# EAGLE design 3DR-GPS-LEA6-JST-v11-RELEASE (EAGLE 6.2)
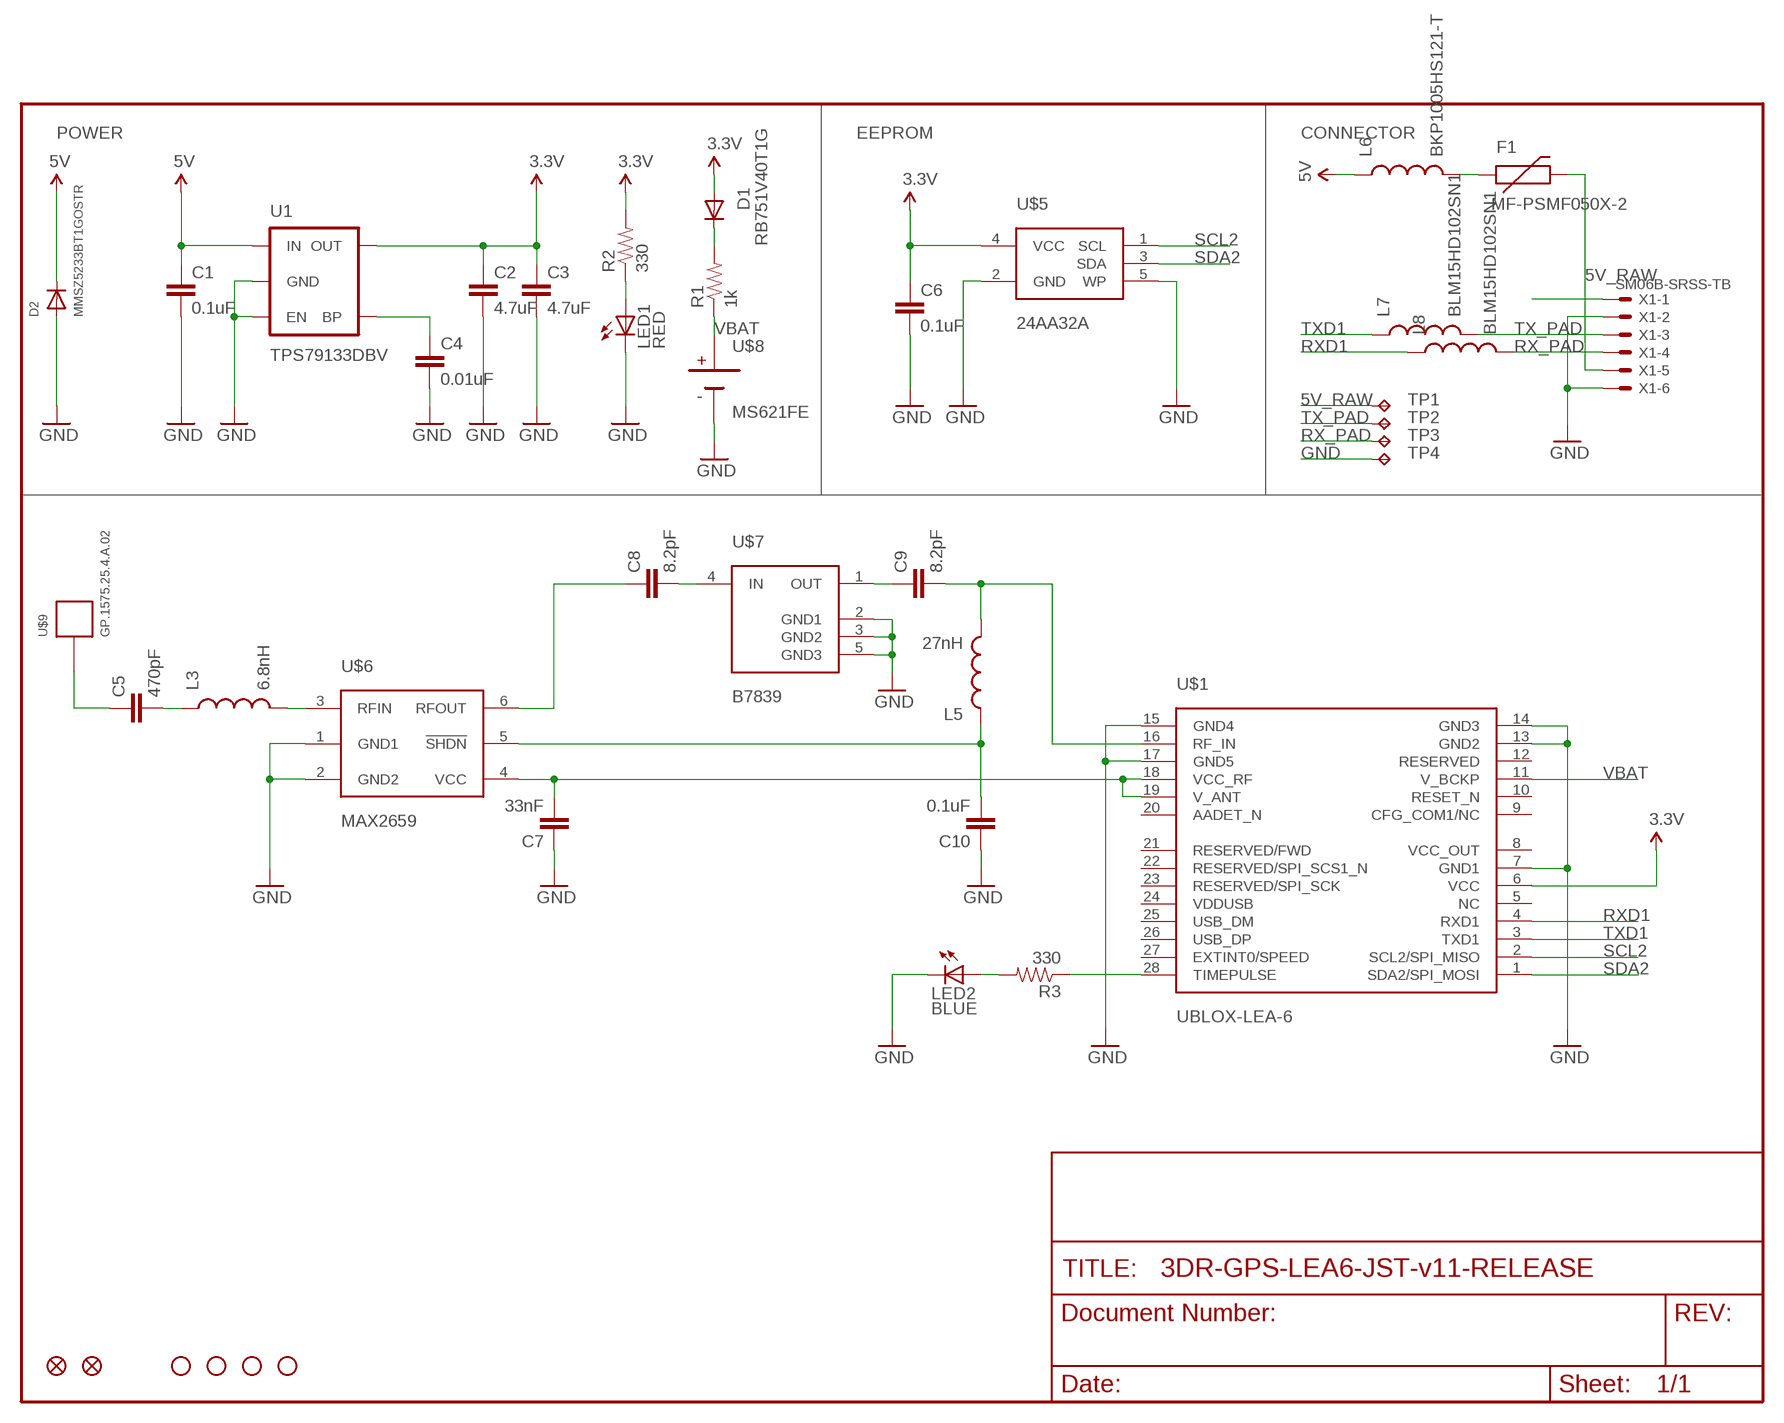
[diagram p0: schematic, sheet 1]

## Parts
C1  0.1uF  CAP0402-CAP  [0402-CAP]
C2  4.7uF  CAP0805  [0805]
C3  4.7uF  CAP0805  [0805]
C4  0.01uF  CAP0402-CAP  [0402-CAP]
C5  470pF  CAP0402-CAP  [0402-CAP]
C6  0.1uF  CAP0402-CAP  [0402-CAP]
C7  33nF  CAP0402-CAP  [0402-CAP]
C8  8.2pF  CAP0402-CAP  [0402-CAP]
C9  8.2pF  CAP0402-CAP  [0402-CAP]
C10  0.1uF  CAP0402-CAP  [0402-CAP]
D1  RB751V40T1G  DIODESOD  [SOD-323]
D2  MMSZ5233BT1GOSTR  DIODESOD-123  [SOD-123]
F1  MF-PSMF050X-2  PTC  [0805]
JP1  FIDUCIAL1X2  [FIDUCIAL-1X2]
JP2  FIDUCIAL1X2  [FIDUCIAL-1X2]
JP3  STAND-OFF  [STAND-OFF]
JP4  STAND-OFF  [STAND-OFF]
JP5  STAND-OFF  [STAND-OFF]
JP6  STAND-OFF  [STAND-OFF]
L3  6.8nH  INDUCTOR0402  [C0402]
L5  27nH  INDUCTOR0402  [C0402]
L6  BKP1005HS121-T  INDUCTOR0402  [0402-IND]
L7  BLM15HD102SN1  INDUCTOR0402  [0402-IND]
L8  BLM15HD102SN1  INDUCTOR0402  [0402-IND]
LED1  RED  LED0603  [LED-0603]
LED2  BLUE  LED0603  [LED-0603]
R1  1k  RESISTOR0402-RES  [0402-RES]
R2  330  RESISTOR0402-RES  [0402-RES]
R3  330  RESISTOR0402-RES  [0402-RES]
TP1  TPTP20SQ  [TP20SQ]
TP2  TPTP20SQ  [TP20SQ]
TP3  TPTP20SQ  [TP20SQ]
TP4  TPTP20SQ  [TP20SQ]
U1  TPS79133DBV  V_REG_LDOSMD  [SOT23-5]
U$1  UBLOX-LEA-6  [UBLOX-LEA-6]
U$5  24AA32A  [SOT23-5]
U$6  MAX2659  [UDFN-6]
U$7  B7839  [QCS5E]
U$8  MS621FE  [MS621FE]
U$9  GP.1575.25.4.A.02  [GP.1575.25.4.A.02]
X1  SM06B-SRSS-TB  [SM06B-SRSS-TB]

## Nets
3.3V: C2.1 C3.1 C6.1 D1.2(A) R2.2 U1.5(OUT) U$1.6(VCC) U$5.4(VCC)
5V: C1.1 D2.C L6.1 U1.1(IN)
5V_RAW: F1.2 TP1.TP X1.5
GND: C1.2 C2.2 C3.2 C4.2 C6.2 C7.1 C10.1 D2.A LED1.C LED2.C TP4.TP U1.2(GND) U1.3(EN) U$1.7(GND1) U$1.13(GND2) U$1.14(GND3) U$1.15(GND4) U$1.17(GND5) U$5.2(GND) U$5.5(WP) U$6.1(GND1) U$6.2(GND2) U$7.2(GND1) U$7.3(GND2) U$7.5(GND3) U$8.2(NEG) X1.2 X1.6
N$1: L3.2 U$6.3(RFIN)
N$2: C4.1 U1.4(BP)
N$3: C5.2 L3.1
N$4: C8.2 U$7.4(IN)
N$5: R3.1 U$1.28(TIMEPULSE)
N$6: C9.1 U$7.1(OUT)
N$7: C7.2 U$1.18(VCC_RF) U$1.19(V_ANT) U$6.4(VCC)
N$8: C8.1 U$6.6(RFOUT)
N$9: C10.2 L5.1 U$6.5(!SHDN)
N$10: C5.1 U$9.1(PIN)
N$11: C9.2 L5.2 U$1.16(RF_IN)
N$12: D1.1(C) R1.2
N$13: LED1.A R2.1
N$14: X1.1
N$15: LED2.A R3.2
N$16: F1.1 L6.2
RX_PAD: L8.2 TP3.TP X1.4
RXD1: L8.1 U$1.4(RXD1)
SCL2: U$1.2(SCL2/SPI_MISO) U$5.1(SCL)
SDA2: U$1.1(SDA2/SPI_MOSI) U$5.3(SDA)
TX_PAD: L7.2 TP2.TP X1.3
TXD1: L7.1 U$1.3(TXD1)
VBAT: R1.1 U$1.11(V_BCKP) U$8.1(POS)
Unconnected: U$1.5(NC) U$1.8(VCC_OUT) U$1.9(CFG_COM1/NC) U$1.10(RESET_N) U$1.12(RESERVED) U$1.20(AADET_N) U$1.21(RESERVED/FWD) U$1.22(RESERVED/SPI_SCS1_N) U$1.23(RESERVED/SPI_SCK) U$1.24(VDDUSB) U$1.25(USB_DM) U$1.26(USB_DP) U$1.27(EXTINT0/SPEED)

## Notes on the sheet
- POWER | EEPROM | CONNECTOR

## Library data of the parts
C1-C10 = SparkFun:CAP: Capacitor
D1 = SparkFun:DIODE: Diode
D2 = adafruit:DIODE: Diode
F1 = 3DRobotics:PTC: Resettable Fuse PTC; DATASHEET: http://www.bourns.com/data/global/PDFs/mfpsmf.pdf; LINK: http://parts.digikey.com/1/parts/1323493-fuse-ptc-resettable-smd-0805-mf-psmf050x-2.html; MFGPN: MF-PSMF050X-2
JP1 JP2 = SparkFun:FIDUCIAL: Fiducial Alignment Points
JP3-JP6 = SparkFun:STAND-OFF: Stand Off
L3 L5 = SparkFun:INDUCTOR: Inductors
L6-L8 = pixhawk2:INDUCTOR: Inductors
LED1 LED2 = SparkFun:LED: LEDs
R1-R3 = SparkFun:RESISTOR: Resistor
TP1-TP4 = testpad:TP: Test pad
U1 = SparkFun:V_REG_LDO: Voltage Regulator LDO Standard 150mA LDO voltage regulator in SOT-23 layout. Micrel part MIC5205. BP (by-pass) pin is used to lower output noise with 470pF cap.
U$1 = 3DRobotics:UBLOX-LEA-6: u-blox LEA-6 GPS Module The LEA-6 module series is a family of stand-alone GPS receivers featuring the high performance u-blox 6 positioning engine. These versatile receivers feature an extensive and flexible range of functionality, connectivity and cost savings options. LEA-6 modules maintain the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; DATASHEET: http://www.u-blox.com/images/downloads/Product_Docs/LEA-6_DataSheet_%28GPS.G6-HW-09004%29.pdf; LINK: http://www.u-blox.com/en/gps-modules/pvt-modules/lea-6-family.html; MFGPN: LEA-6
U$5 = 3DRobotics:24AA32A: Microchip 24AA32A 32K I2C EEPROM The Microchip Technology Inc. 24AA32A/24LC32A (24XX32A*) is a 32 Kbit Electrically Erasable PROM. The device is organized as a single block of 4K x 8-bit memory with a 2-wire serial interface. Low-voltage design permits operation down to 1.7V, with standby and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; DATASHEET: http://ww1.microchip.com/downloads/en/DeviceDoc/21713L.pdf; LINK: http://www.microchip.com/wwwproducts/Devices.aspx?dDocName=en010787; MFGPN: 24AA32A
U$6 = 3DRobotics:MAX2659: MAX2659 GPS/GNSS Low-Noise Amplifier The MAX2659 high-gain, low-noise amplifier (LNA) is designed for GPS, Galileo, and GLONASS applications. Designed in Maxim?s advanced SiGe process, the device achieves a 20.5dB gain and an ultra-low-noise figure of 0.8dB while maximizing the input-referred 1dB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; DATASHEET: http://datasheets.maxim-ic.com/en/ds/MAX2659.pdf; LINK: http://www.maxim-ic.com/datasheet/index.mvp/id/5299; MFGPN: MAX2659
U$7 = 3DRobotics:B7839: EPCOS B7839 SAW Rx Filter; DATASHEET: http://www.epcos.com/inf/40/ds/mc/B7839.pdf; MFGPN: B7839
U$8 = 3DRobotics:MS621FE: SEIKO 6.8mm Rechargeable 3V lithium battery; DATASHEET: http://speed.sii.co.jp/data/file_PRODUCT_MASTER_50112_TITLE_IMAGESP.pdf; LINK: http://search.digikey.com/us/en/products/MS621FE-FL11E/728-1057-ND/1889208; MFGPN: MS621FE
U$9 = 3DRobotics:GP.1575.25.4.A.02: Taoglas GP.1575.25.4.A.02 4mm thick GPS Patch Antenna, 1575MHz; DATASHEET: http://www.taoglas.com/images/product_images/original_images/GP.1575.25.4.A.02%20GPS%20Patch%20Antenna%201575MHz%20190410.pdf; LINK: http://www.taoglas.com/antennas/GPS-GLONASS_Antennas/Internal_GPS_-_Passive_Ceramic_Patch_Antennas/; MFGPN: GP.1575.25.4.A.02
X1 = con-jst2:?M06B-SRSS-TB: Disconnectable Crimp style connector, 1.0mm pitch 6 contacts

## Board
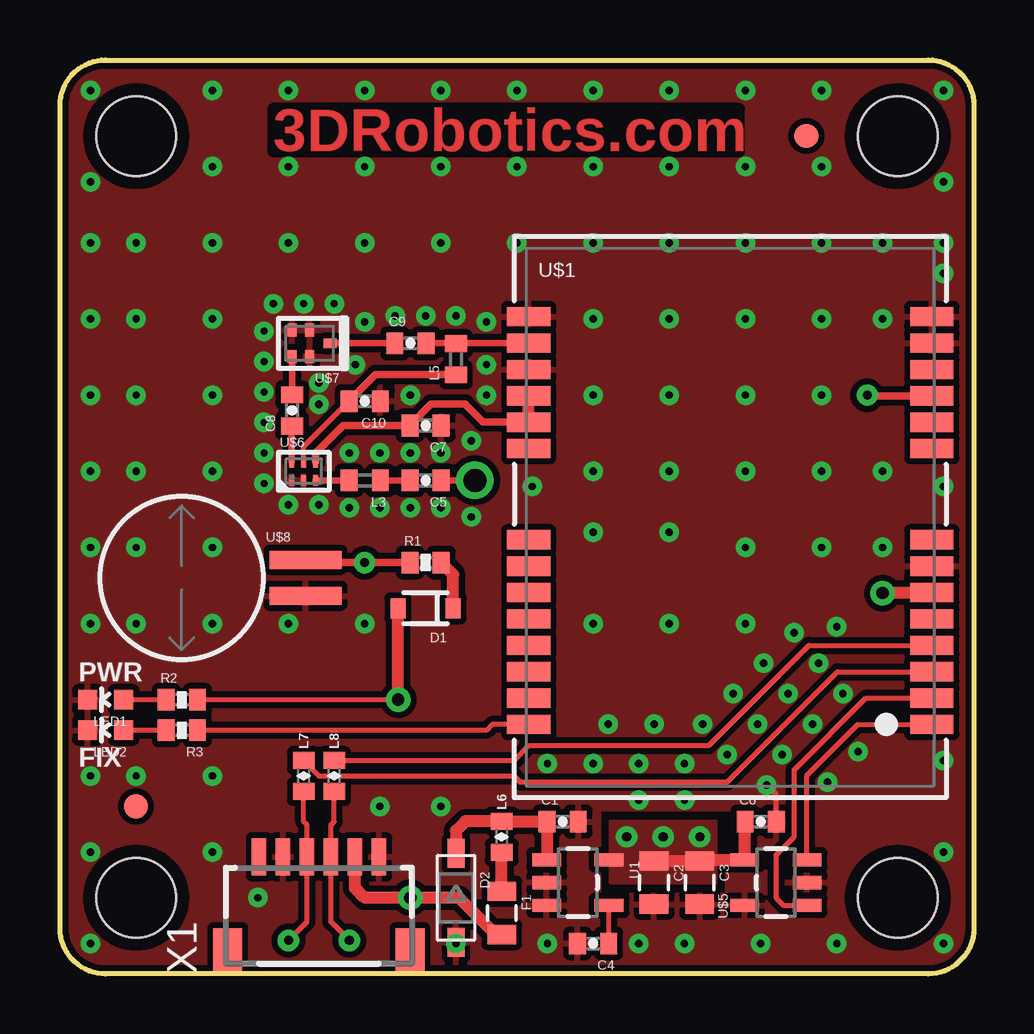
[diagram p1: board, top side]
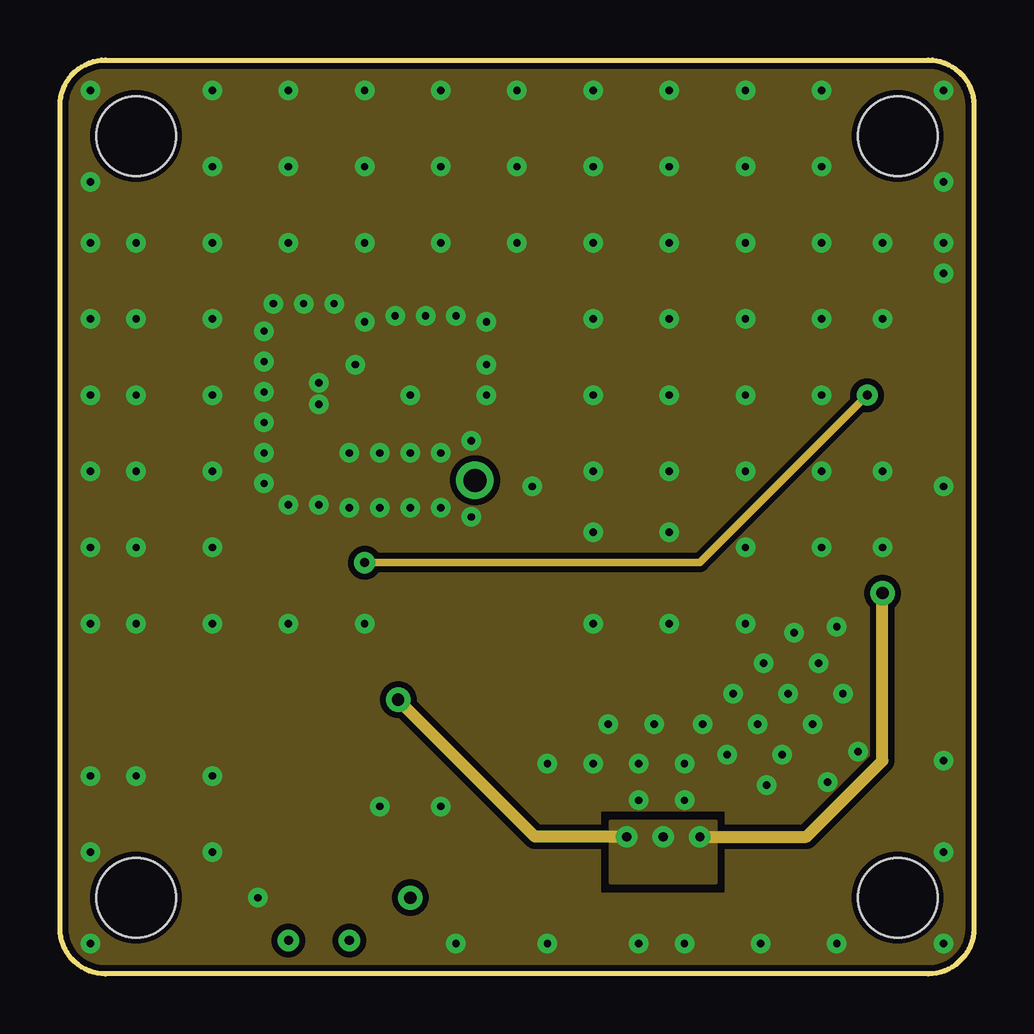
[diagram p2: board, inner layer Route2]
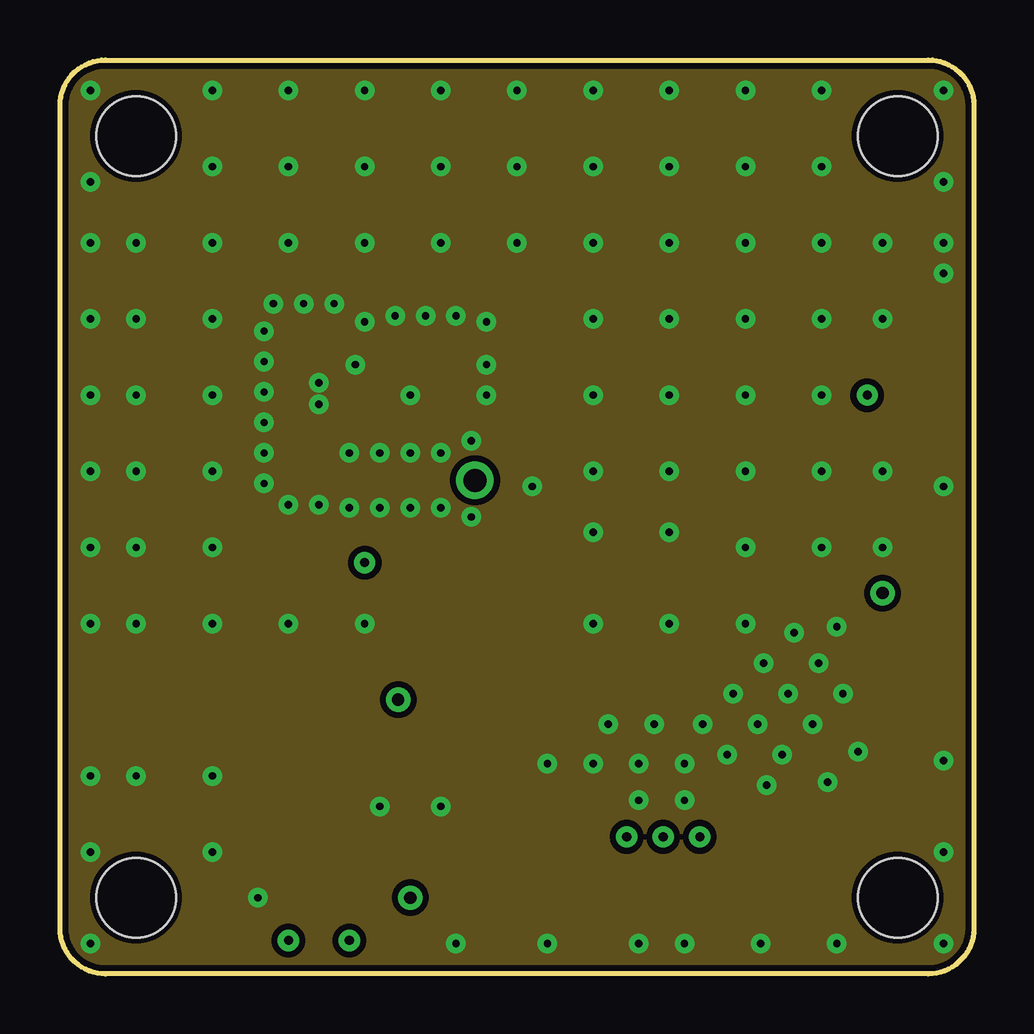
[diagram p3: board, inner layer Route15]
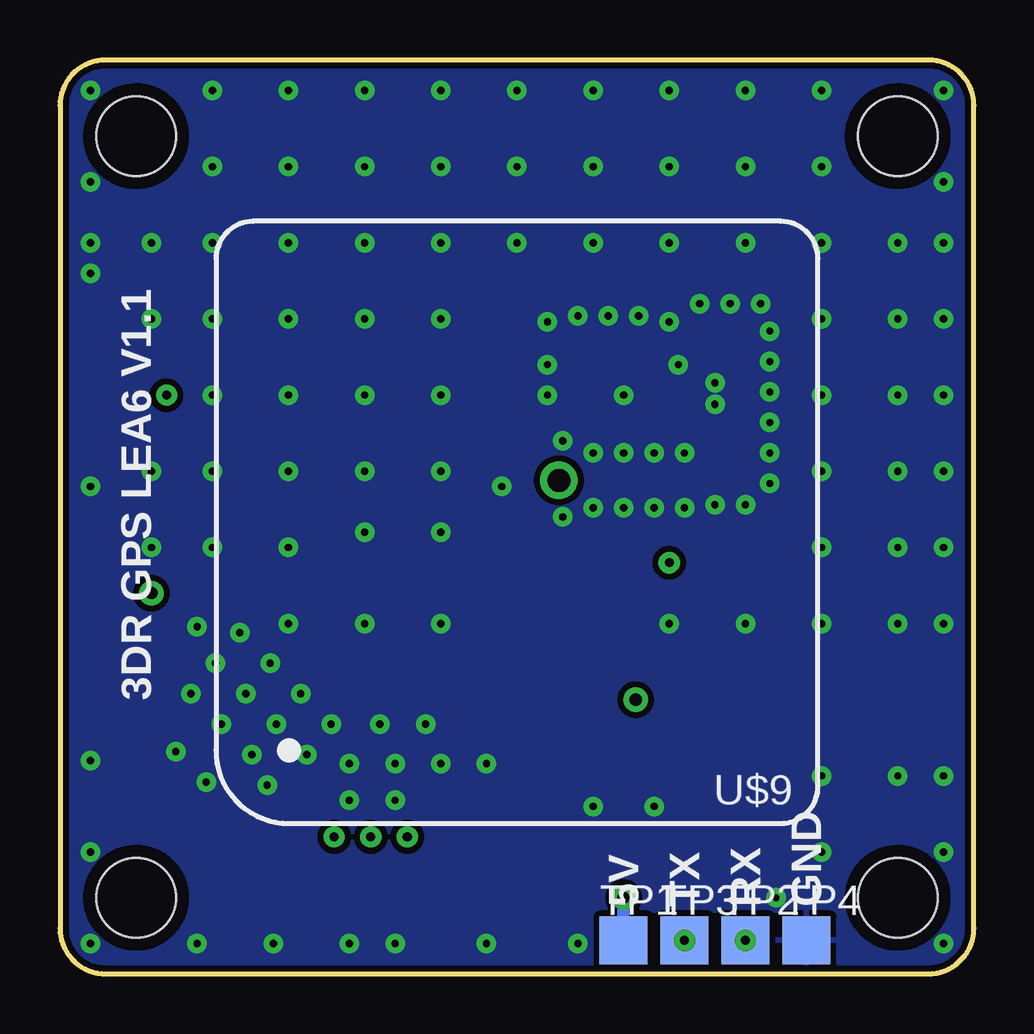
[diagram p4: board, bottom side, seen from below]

Size 38.1 x 38.1 mm. Coordinates in mm from the lower left corner, seen from the top.
Outline: 1.91,0 arc-90 0,1.91 0,36.2 arc-90 1.91,38.1 36.2,38.1 arc-90 38.1,36.2 38.1,1.91 arc-90 36.2,0 1.91,0
Copper layers (1*2*15*16): Top 0.035mm / dielectric 0.5mm / Route2 0.035mm / dielectric 0.5mm / Route15 0.035mm / dielectric 0.5mm / Bottom 0.035mm
Design rules: minimum track width 7mil, minimum drill 10mil, track to track 7mil, track to pad 7mil, pad to pad 7mil, via to via 7mil, smd to smd 0mil, copper to edge 10mil, drill to drill 8mil, minimum pad ring 12mil, minimum via ring 10mil, stop-mask expansion 4mil, vias tented up to drill 25mil, thermal gap 10mil

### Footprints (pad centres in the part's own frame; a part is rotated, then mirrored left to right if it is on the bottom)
0402-CAP = smd 0.7 x 0.9: 1 -0.65,0; 2 0.65,0
0805 = smd 0.8 x 1.2: 1 -0.9,0; 2 0.9,0
SOD-323 = smd 0.63 x 0.83: 1 -1.15,0; 2 1.15,0
SOD-123 = smd 1.2 x 0.7: A 1.85,0; C -1.85,0
FIDUCIAL-1X2 = smd 1 x 1: 1 0,0
STAND-OFF = hole 3.302: 0,0
C0402 = smd 0.7 x 0.9: 1 -0.65,0; 2 0.65,0
0402-IND = smd 0.7 x 0.9: 1 -0.65,0; 2 0.65,0
LED-0603 = smd 0.8 x 0.8: A 0,-0.75; C 0,0.75
0402-RES = smd 0.7 x 0.9: 1 -0.65,0; 2 0.65,0
TP20SQ = smd 2 x 2: TP 0,0
SOT23-5 = smd 0.55 x 1.2: 1 -0.95,-1.3; 2 0,-1.3; 3 0.95,-1.3; 4 0.95,1.3; 5 -0.95,1.3
UBLOX-LEA-6 = smd 1.8 x 0.8: 1 8.4,-8.65; 2 8.4,-7.55; 3 8.4,-6.45; 4 8.4,-5.35; 5 8.4,-4.25; 6 8.4,-3.15; 7 8.4,-2.05; 8 8.4,-0.95; 9 8.4,2.85; 10 8.4,3.95; 11 8.4,5.05; 12 8.4,6.15; 13 8.4,7.25; 14 8.4,8.35; 15 -8.4,8.35; 16 -8.4,7.25; 17 -8.4,6.15; 18 -8.4,5.05; 19 -8.4,3.95; 20 -8.4,2.85; 21 -8.4,-0.95; 22 -8.4,-2.05; 23 -8.4,-3.15; 24 -8.4,-4.25; 25 -8.4,-5.35; 26 -8.4,-6.45; 27 -8.4,-7.55; 28 -8.4,-8.65
UDFN-6 = smd 0.2 x 0.45: 1 -0.5,-0.375; 2 0,-0.375; 3 0.5,-0.375; 4 0.5,0.375; 5 0,0.375; 6 -0.5,0.375
QCS5E = smd 0.55 x 0.38: 1 -0.85,0 | smd 0.38 x 0.55: 2 0,-0.55; 3 0.735,-0.55; 4 0.735,0.55; 5 0,0.55
MS621FE = smd 3 x 0.75: 1 5.15,0.75; 2 5.15,-0.75
GP.1575.25.4.A.02 = drill 0.95: 1 -1.75,-1.75
SM06B-SRSS-TB = smd 0.6 x 1.55: 1 -2.5,2.975; 2 -1.5,2.975; 3 -0.5,2.975; 4 0.5,2.975; 5 1.5,2.975; 6 2.5,2.975 | smd 1.2 x 1.8: FIT@1 -3.8,-0.9; FIT@2 3.8,-0.9

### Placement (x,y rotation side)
C1  20.95,6.35 0 top
C2  24.77,3.81 270 top
C3  26.67,3.81 270 top
C4  22.23,1.27 180 top
C5  15.24,20.57 180 top
C6  29.21,6.35 0 top
C7  15.24,22.86 180 top
C8  9.68,23.5 90 top
C9  14.61,26.29 0 top
C10  12.7,23.88 180 top
D1  15.24,15.24 180 top
D2  16.51,3.17 270 top
F1  18.41,2.54 270 top
JP1  31.11,34.92 0 top
JP2  3.17,6.99 0 top
JP3  3.17,3.17 0 top
JP4  3.17,34.92 0 top
JP5  34.92,34.92 0 top
JP6  34.92,3.17 0 top
L3  12.7,20.57 180 top
L5  16.51,25.63 90 top
L6  18.41,5.71 270 top
L7  10.16,8.26 270 top
L8  11.43,8.26 270 top
LED1  1.91,11.43 90 top
LED2  1.91,10.16 90 top
R1  15.24,17.14 0 top
R2  5.08,11.43 0 top
R3  5.08,10.16 180 top
TP1  14.61,1.4 0 bottom
TP2  9.53,1.4 0 bottom
TP3  12.06,1.4 0 bottom
TP4  6.99,1.4 0 bottom
U1  21.59,3.81 270 top
U$1  27.94,19.05 0 top
U$5  29.84,3.81 90 top
U$6  10.16,20.95 0 top
U$7  10.41,26.29 180 top
U$8  5.08,16.51 0 top
U$9  19.05,18.82 180 bottom
X1  10.79,1.91 0 top

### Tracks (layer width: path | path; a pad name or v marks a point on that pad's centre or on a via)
3.3V  (via drill 0.38, 0.51)
  Top 0.203: v14.1,11.43 R2.2
  Top 0.508: 24.71,4.76 C2.1 C3.1 26.72,4.76 U$5.4 28.56,4.78 C6.1 | U$1.6 34.31,15.9 v34.29,15.88 | v14.1,11.43 D1.2
  Route2 0.508: v34.29,15.88 34.29,8.89 31.11,5.71 v26.67,5.71 | v23.62,5.71 19.81,5.71 v14.1,11.43
  other vias: 25.15,5.71
  pour Top (isolate 0.254, no thermals): 22.99,3.81 22.99,6.35 27.3,6.35 27.3,3.81
  pour Route2 (isolate 0.254): 22.99,3.81 22.99,6.35 27.3,6.35 27.3,3.81
5V
  Top 0.508: U1.1 20.3,4.78 C1.1 18.43,6.35 L6.1 16.91,6.37 16.51,5.97 D2.C
5V_RAW  (via drill 0.51)
  Top 0.508: X1.5 12.29,3.58 12.7,3.17 v14.61,3.17 16.64,3.17 18.17,1.64 F1.2
  Bottom 0.508: TP1.TP v14.61,3.17
GND  (via drill 0.3)
  Top 0.203: C6.2 29.86,7.48 v29.46,7.87
  other vias: 20.32,1.27 26.04,1.27 32.38,1.27 29.21,1.27 33.27,9.27 1.27,8.26 36.83,5.08 36.83,8.89 12.7,14.61 3.17,14.61 1.27,20.95 9.53,14.61 1.27,24.13 1.27,27.3 3.17,30.48 1.27,33.02 6.35,33.66 6.35,36.83 9.53,36.83 12.7,36.83 15.88,36.83 19.05,36.83 22.23,36.83 25.4,36.83 28.57,36.83 36.83,33.02 36.83,29.21 36.83,20.32 20.32,8.76 22.23,8.76 24.13,8.76 26.04,8.76 27.81,9.14 29.08,10.41 31.62,12.95 30.35,11.68 32.64,11.68 31.37,10.41 30.1,9.14 26.04,7.24 24.13,7.24 13.34,6.99 1.27,36.83 36.83,36.83 36.83,1.27 1.27,1.27 15.88,6.99 16.51,1.27 32,8 22.86,10.41 24.77,10.41 26.8,10.41 28.07,11.68 29.34,12.95 30.61,14.22 32.38,14.48 17.78,25.4 17.78,24.13 17.78,27.18 16.51,27.43 15.24,27.43 13.97,27.43 12.7,27.18 11.43,27.94 10.16,27.94 8.89,27.94 8.51,26.8 8.51,25.53 8.51,24.26 10.79,23.75 8.51,22.99 8.51,21.72 10.79,24.64 8.51,20.45 9.53,19.56 10.79,19.56 12.06,19.43 13.34,19.43 14.61,19.43 15.88,19.43 14.61,21.72 15.88,21.72 31.75,36.83 6.35,30.48 9.53,33.66 12.7,33.66 15.88,33.66 19.05,33.66 22.23,33.66 25.4,33.66 28.57,33.66 31.75,33.66 9.53,30.48 12.7,30.48 15.88,30.48 19.05,30.48 22.23,30.48 25.4,30.48 28.57,30.48 31.75,30.48 36.83,30.48 1.27,30.48 1.27,5.08 3.17,27.3 3.17,24.13 1.27,17.78 3.17,17.78 3.17,8.26 24.13,1.27 34.29,30.48 34.29,27.3 31.75,27.3 28.57,27.3 25.4,27.3 22.23,27.3 22.23,24.13 25.4,24.13 28.57,24.13 31.75,24.13 34.29,20.95 31.75,20.95 28.57,20.95 25.4,20.95 22.23,20.95 34.29,17.78 31.75,17.78 28.57,17.78 25.4,18.41 22.23,18.41 28.57,14.61 25.4,14.61 1.27,14.61 3.17,20.95 6.35,8.26 12.32,25.4 6.35,14.61 6.35,20.95 6.35,17.78 6.35,27.3 6.35,24.13 13.34,21.72 12.06,21.72 14.61,24.13 17.14,22.23 17.14,19.05 19.68,20.32 8.26,3.17 22.23,14.61 6.35,5.08
  pour Route15 (isolate 0.254): 0,0 0,41.91 38.1,41.91 38.1,0
  pour Top (isolate 0.254): 22.23,0 22.23,3.3 27.81,3.3 27.81,6.99 39.37,6.99 39.37,0
  pour Top (isolate 0.254): 22.48,0 22.48,39.37 0,39.37 0,0
  pour Bottom (isolate 0.254): 0,0 0,39.37 0,43.18 38.1,43.18 38.1,0
  pour Route2 (isolate 0.254): 0,0 22.48,0 22.48,40.64 0,40.64
  pour Top (isolate 0.254): 39.37,6.86 22.23,6.86 22.23,39.37 39.37,39.37
  pour Route2 (isolate 0.254): 22.48,0 22.48,3.3 27.81,3.3 27.81,6.86 22.48,6.86 22.48,40.64 38.1,40.64 38.1,0
N$1
  Top 0.265: L3.2 U$6.3
N$2
  Top 0.203: U1.4 22.89,1.28 C4.1
N$3
  Top 0.265: L3.1 C5.2
N$4
  Top 0.265: U$7.4 C8.2
N$5
  Top 0.203: R3.1 17.78,10.16 18.02,10.4 U$1.28
N$6
  Top 0.265: U$7.1 C9.1
N$7
  Top 0.305: U$1.19 17.64,23 16.89,23.75 15.48,23.75 C7.2 11.81,22.86 10.66,21.71 U$6.4
  Top 0.508: U$1.19 U$1.18
N$8
  Top 0.265: U$6.6 9.66,22.83 C8.1
N$9
  Top 0.203: U$6.5 10.16,21.99 C10.2
  Top 0.305: L5.1 13.15,24.98 C10.2
N$10
  Top 0.265: C5.1 U$9.1
N$11
  Top 0.265: C9.2 16.35,26.29 L5.2 16.68,26.3 U$1.16
N$12
  Top 0.508: 15.88,17.13 R1.2 16.39,16.64 D1.1
N$13
  Top 0.203: R2.1 LED1.A
N$15
  Top 0.203: R3.2 LED2.A
N$16
  Top 0.508: F1.1 L6.2
RX_PAD  (via drill 0.38)
  Top 0.203: TP3.TP 11.29,2.17 X1.4 11.29,6.21 11.43,6.35 L8.2
  other vias: 12.06,1.4
RXD1
  Top 0.203: U$1.4 31.23,13.7 27.05,9.53 19.56,9.53 18.94,8.9 L8.1
SCL2
  Top 0.203: U$1.2 33.6,11.5 30.61,8.51 30.61,5.71 29.84,4.95 29.84,3.17 30.16,2.86 U$5.1
SDA2
  Top 0.203: U$1.1 33.26,10.4 31.14,8.29 U$5.3
TX_PAD  (via drill 0.38)
  Top 0.203: TP2.TP 10.29,2.17 X1.3 10.29,6.21 10.16,6.35 L7.2
  other vias: 9.53,1.4
TXD1
  Top 0.203: U$1.3 32.41,12.6 27.81,8 19.18,8 18.92,8.26 10.79,8.26 10.16,8.89 L7.1
VBAT  (via drill 0.38)
  Top 0.305: U$1.11 33.69,24.1 v33.66,24.13 | R1.1 v12.7,17.14 10.35,17.14 U$8.1
  Route2 0.305: v12.7,17.14 26.67,17.14 v33.66,24.13

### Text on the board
Top: 3DRobotics.com
tPlace: PWR | FIX
bPlace: 3DR GPS LEA6 V1.1 | GND | RX | TX | 5V
tStop: 3DRobotics.com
